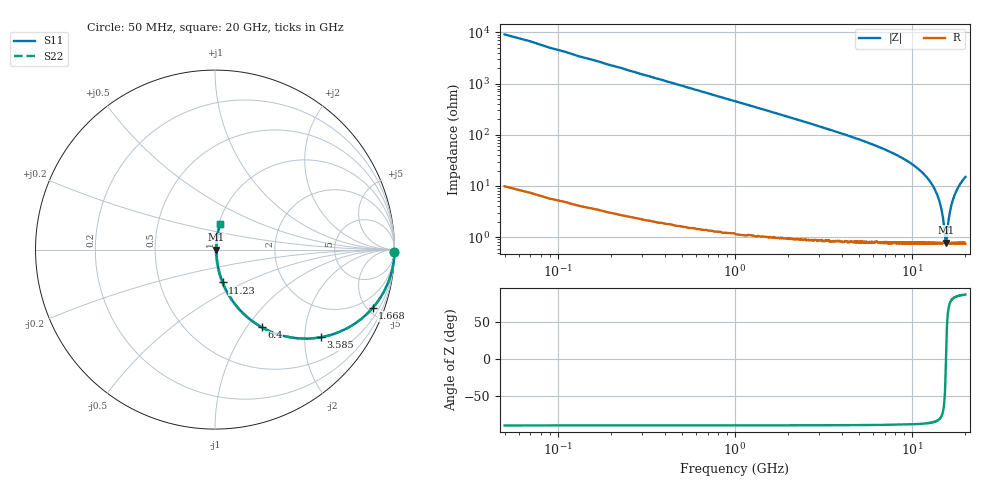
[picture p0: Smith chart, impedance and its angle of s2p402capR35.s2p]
! AVX Thin Film Operation		Date: September 2011
! Description: Accu-P® Series, Thin Film, SMD, RF Capacitor
! Part Number: 04021JR35ZBW/STR
! 50 MHz  -  20 GHz
! Serial Measurements
# MHZ S MA R 50
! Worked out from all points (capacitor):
!   1000 points, 50 MHz to 20 GHz, reference 50 ohm
!   read as one part in series: C = 349 fF near 149.8 MHz
!   lowest |Z| = 785 mohm at 15.53 GHz (marker M1)
!   series resonance near 15.54 GHz, so ESL is about 300 pH
!   S11 on the Smith chart (normalised r, x): 50 MHz: open; 1.668 GHz: 1.03, -5.39; 3.585 GHz: 1.02, -2.40; 6.4 GHz: 1.02, -1.18; 11.23 GHz: 1.02, -0.39; 20 GHz: 1.02, +0.30
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50  1 -0.6  0.011 89.3  0.011 89.3  1 -0.6
249.7  0.998 -3.1  0.055 86.8  0.055 86.8  0.998 -3.1
509.309  0.994 -6.4  0.111 83.5  0.111 83.5  0.994 -6.4
988.589  0.976 -12.3  0.213 77.5  0.213 77.5  0.976 -12.3
1667.568  0.936 -20.3  0.347 69.5  0.347 69.5  0.936 -20.3
3384.985  0.785 -37.9  0.614 51.8  0.614 51.8  0.785 -37.9
3584.685  0.766 -39.6  0.638 50.0  0.638 50.0  0.766 -39.6
6400.45  0.505 -58.9  0.856 30.3  0.856 30.3  0.505 -58.9
6700  0.481 -60.5  0.87 28.7  0.87 28.7  0.481 -60.5
10034.99  0.254 -73.6  0.96 14.7  0.96 14.7  0.254 -73.6
11233.18  0.188 -76.9  0.975 10.9  0.975 10.9  0.188 -76.9
13350  0.088 -80.0  0.989 5.1  0.989 5.1  0.088 -80.0
14068.92  0.058 -79.2  0.991 3.3  0.991 3.3  0.058 -79.2
14628.08  0.036 -75.8  0.992 2.0  0.992 2.0  0.036 -75.8
15047.45  0.02 -66.7  0.992 1.1  0.992 1.1  0.02 -66.7
15406.91  0.008972 -32.1  0.992 0.3  0.992 0.3  0.008972 -32.1
15526.73  0.00758 -2.3  0.992 0.0  0.992 0.0  0.00758 -2.3
15666.52  0.00902 32.6  0.992 -0.3  0.992 -0.3  0.00902 32.6
16105.86  0.022 68.9  0.992 -1.2  0.992 -1.2  0.022 68.9
16684.99  0.042 77.3  0.992 -2.4  0.992 -2.4  0.042 77.3
17983.03  0.085 80.0  0.989 -4.9  0.989 -4.9  0.085 80.0
20000  0.147 78.6  0.982 -8.4  0.982 -8.4  0.147 78.6
